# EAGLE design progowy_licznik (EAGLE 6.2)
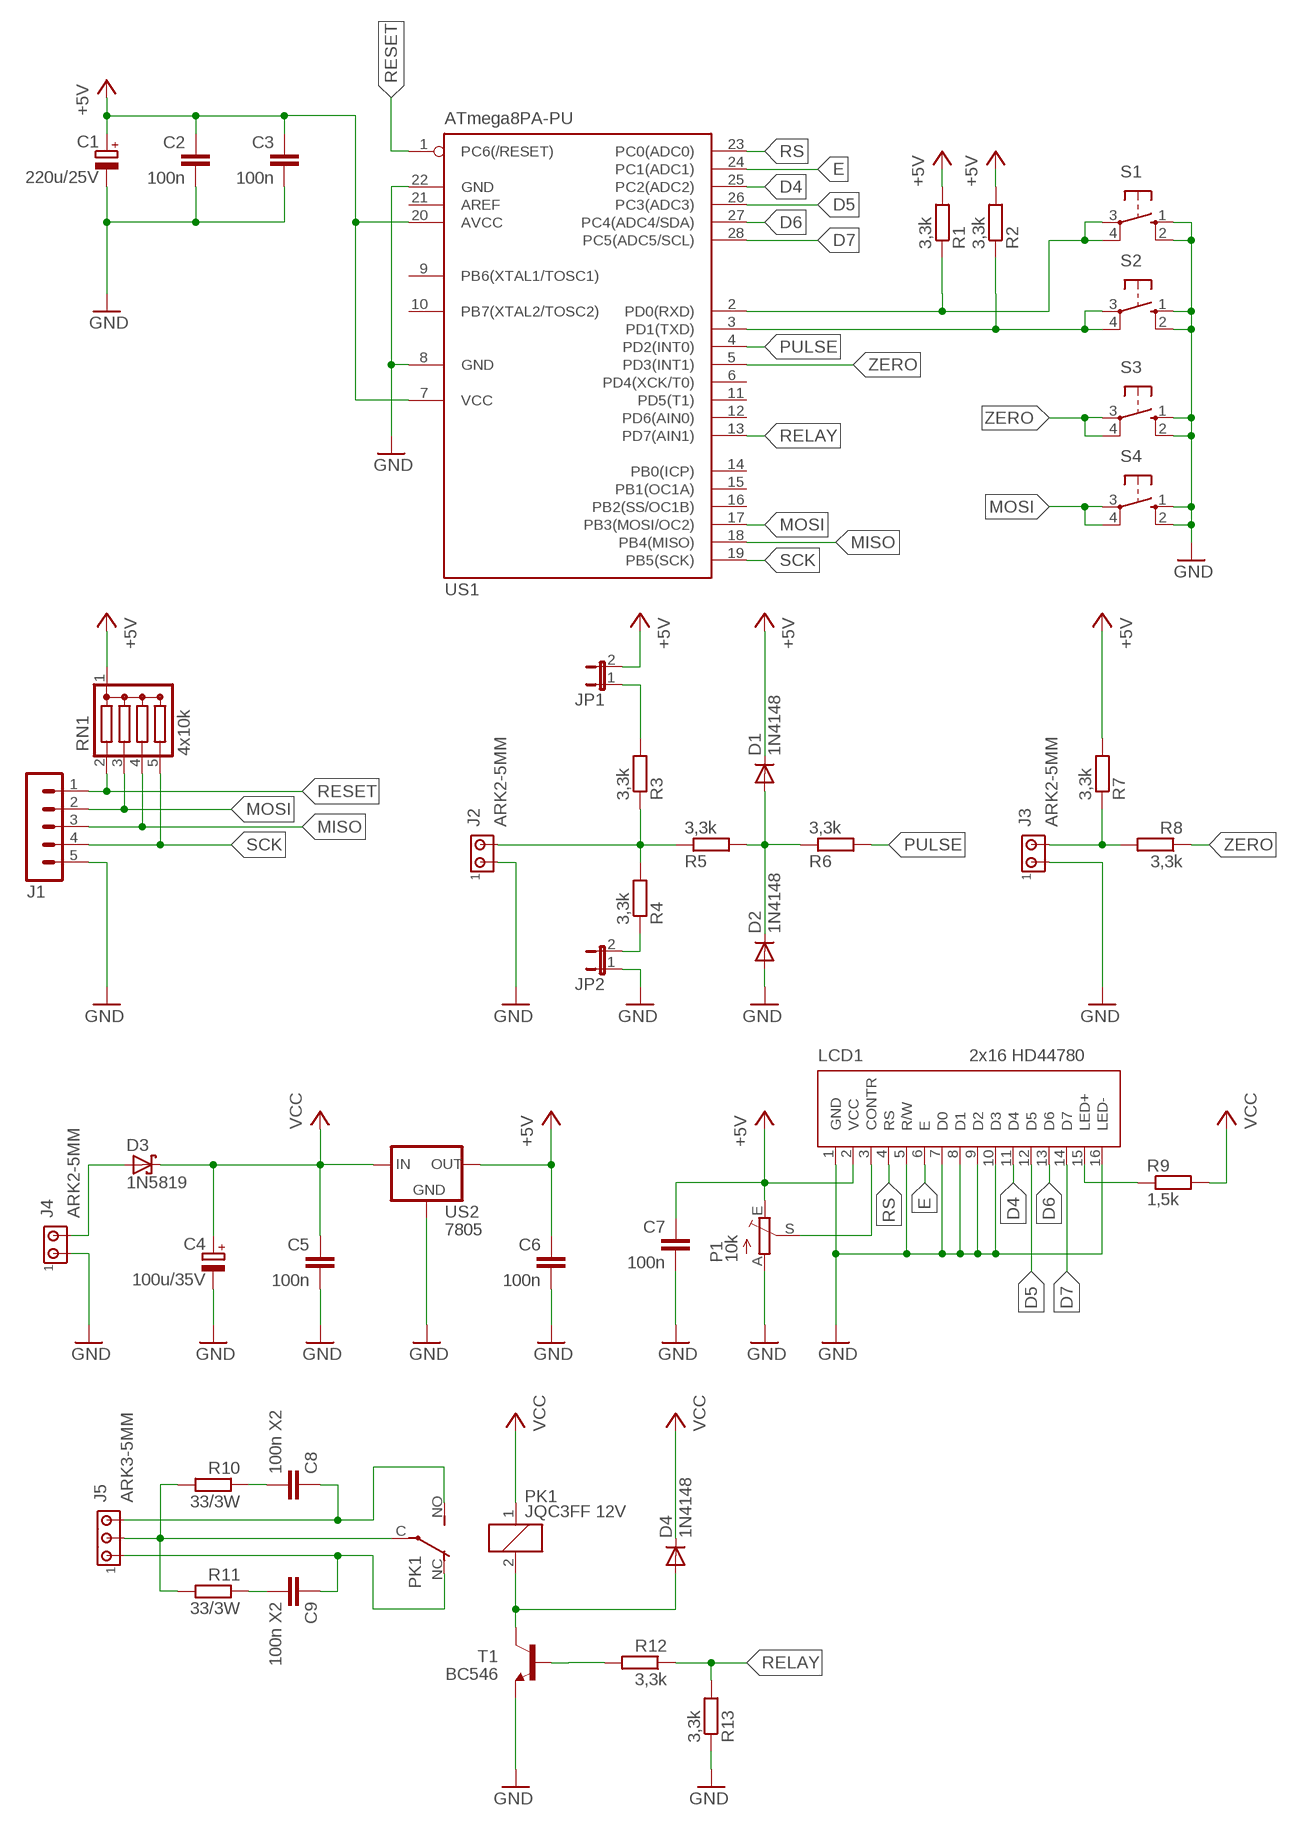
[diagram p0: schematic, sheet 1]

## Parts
C1  220u/25V  CPOL-EUE2.5-7  [E2,5-7]
C2  100n  C-EU050-025X075  [C050-025X075]
C3  100n  C-EU050-025X075  [C050-025X075]
C4  100u/35V  CPOL-EUE2.5-7  [E2,5-7]
C5  100n  C-EU050-025X075  [C050-025X075]
C6  100n  C-EU050-025X075  [C050-025X075]
C7  100n  C-EU050-025X075  [C050-025X075]
C8  100n X2  C-EU102_152-062X184  [C102_152-062X184]
C9  100n X2  C-EU102_152-062X184  [C102_152-062X184]
D1  1N4148  BAT81  [DO34-7]
D2  1N4148  BAT81  [DO34-7]
D3  1N5819  SCHOTTKY-DIODEF126Z12  [F126Z12]
D4  1N4148  BAT81  [DO34-7]
J1  MA05-1  [MA05-1]
J2  ARK2-5MM  [2PIN-5MM]
J3  ARK2-5MM  [2PIN-5MM]
J4  ARK2-5MM  [2PIN-5MM]
J5  ARK3-5MM  [3PIN-5MM]
JP1  JP1E  [JP1]
JP2  JP1E  [JP1]
LCD1  2x16 HD44780  LCD_2X16-NAD-ELEMENTAMI  [LCD_HD44780_2X16_NAD-ELEMENTAMI]
P1  10k  TRIM_EU-CA6V  [CA6V]
PK1  JQC3FF 12V  PK_POJED-JQC-3FG  [PK_POJED_JQC-3FG]
R1  3,3k  R-EU_0207/7  [0207/7]
R2  3,3k  R-EU_0207/7  [0207/7]
R3  3,3k  R-EU_0207/7  [0207/7]
R4  3,3k  R-EU_0207/7  [0207/7]
R5  3,3k  R-EU_0207/7  [0207/7]
R6  3,3k  R-EU_0207/7  [0207/7]
R7  3,3k  R-EU_0207/7  [0207/7]
R8  3,3k  R-EU_0207/7  [0207/7]
R9  1,5k  R-EU_0207/7  [0207/7]
R10  33/3W  R-EU_0617/17  [0617/17]
R11  33/3W  R-EU_0617/17  [0617/17]
R12  3,3k  R-EU_0207/7  [0207/7]
R13  3,3k  R-EU_0207/7  [0207/7]
RN1  4x10k  DRAB_REZ_1X4  [RN-5]
S1  10-XX  [B3F-10XX]
S2  10-XX  [B3F-10XX]
S3  10-XX  [B3F-10XX]
S4  10-XX  [B3F-10XX]
T1  BC546  BC546A  [TO92-EBC]
US1  ATmega8PA-PU  MEGA8-P  [DIL28-3]
US2  7805  78XXL  [78XXL]

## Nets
+5V: C1.+ C2.1 C3.1 C6.1 C7.1 D1.C JP1.2 LCD1.2(VCC) P1.E R1.2 R2.2 R7.2 RN1.1(C) US1.7(VCC) US1.20(AVCC) US2.OUT
D4: LCD1.11(D4) US1.25(PC2(ADC2))
D5: LCD1.12(D5) US1.26(PC3(ADC3))
D6: LCD1.13(D6) US1.27(PC4(ADC4/SDA))
D7: LCD1.14(D7) US1.28(PC5(ADC5/SCL))
E: LCD1.6(E) US1.24(PC1(ADC1))
GND: C1.- C2.2 C3.2 C4.- C5.2 C6.2 C7.2 D2.A J1.5 J2.P$1 J3.P$1 J4.P$1 JP2.1 LCD1.1(GND) LCD1.5(R/W) LCD1.7(D0) LCD1.8(D1) LCD1.9(D2) LCD1.10(D3) LCD1.16(LED-) P1.A R13.1 S1.1(S) S1.2(S1) S2.1(S) S2.2(S1) S3.1(S) S3.2(S1) S4.1(S) S4.2(S1) T1.E US1.8(GND) US1.22(GND) US2.GND
MISO: J1.3 RN1.4 US1.18(PB4(MISO))
MOSI: J1.2 RN1.3 S4.3(P) S4.4(P1) US1.17(PB3(MOSI/OC2))
N$1: LCD1.3(CONTR) P1.S
N$2: J5.P$2 PK1.C(COM) R10.2 R11.2
N$3: JP1.1 R3.2
N$4: JP2.2 R4.1
N$5: R1.1 S1.3(P) S1.4(P1) US1.2(PD0(RXD))
N$6: LCD1.15(LED+) R9.1
N$7: R12.2 T1.B
N$8: D3.A J4.P$2
N$9: D4.A PK1.2 T1.C
N$10: R2.1 S2.3(P) S2.4(P1) US1.3(PD1(TXD))
N$11: C8.1 J5.P$3 PK1.NO
N$12: C9.1 J5.P$1 PK1.NC
N$13: C8.2 R10.1
N$14: C9.2 R11.1
N$15: J3.P$2 R7.1 R8.2
N$20: J2.P$2 R3.1 R4.2 R5.1
N$21: D1.A D2.C R5.2 R6.1
PULSE: R6.2 US1.4(PD2(INT0))
RELAY: R12.1 R13.2 US1.13(PD7(AIN1))
RESET: J1.1 RN1.2 US1.1(PC6(/RESET))
RS: LCD1.4(RS) US1.23(PC0(ADC0))
SCK: J1.4 RN1.5 US1.19(PB5(SCK))
VCC: C4.+ C5.1 D3.C D4.C PK1.1 R9.2 US2.IN
ZERO: R8.1 S3.3(P) S3.4(P1) US1.5(PD3(INT1))
Unconnected: US1.6(PD4(XCK/T0)) US1.9(PB6(XTAL1/TOSC1)) US1.10(PB7(XTAL2/TOSC2)) US1.11(PD5(T1)) US1.12(PD6(AIN0)) US1.14(PB0(ICP)) US1.15(PB1(OC1A)) US1.16(PB2(SS/OC1B)) US1.21(AREF)

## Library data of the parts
C1 C4 = rcl:CPOL-EU: POLARIZED CAPACITOR, European symbol
C2 C3 C5-C9 = rcl:C-EU: CAPACITOR, European symbol
D1 D2 D4 = diode:BAT81: DIODE
D3 = diode:SCHOTTKY-DIODE: Schottky Diode
J1 = zlacza_futrzak:MA05-1: PIN HEADER; OC_FARNELL: unknown; OC_NEWARK: unknown
J2-J4 = zlacza_futrzak:ARK2: ARK 2
J5 = zlacza_futrzak:ARK3: ARK 3 Raster 5mm i 3,5mm
JP1 JP2 = jumper:JP1E: JUMPER
LCD1 = inne_futrzak:LCD_2X16
P1 = pot:TRIM_EU-: POTENTIOMETER
PK1 = inne_futrzak:PK_POJED
R1-R13 = rcl:R-EU_: RESISTOR, European symbol
RN1 = inne_futrzak:DRAB_REZ_1X4
S1-S4 = switch-omron:10-XX: OMRON SWITCH; MPN: B3F-1000; OC_FARNELL: 176432; OC_NEWARK: 36M3542
T1 = transistor-npn:BC546*: NPN Transistor
US1 = atmel:MEGA8-P: MICROCONTROLLER 8 Kbytes FLASH, 1 kbytes SRAM, 512 bytes EEPROM, USART, 4-channel 10 bit ADC, 2-channel 8 bit ADC Pin compatible with Atmega48, ATMega88, ATMega168 Source: avr.lbr; OC_FARNELL: unknown; OC_NEWARK: unknown
US2 = v-reg:78XXL: VOLTAGE REGULATOR

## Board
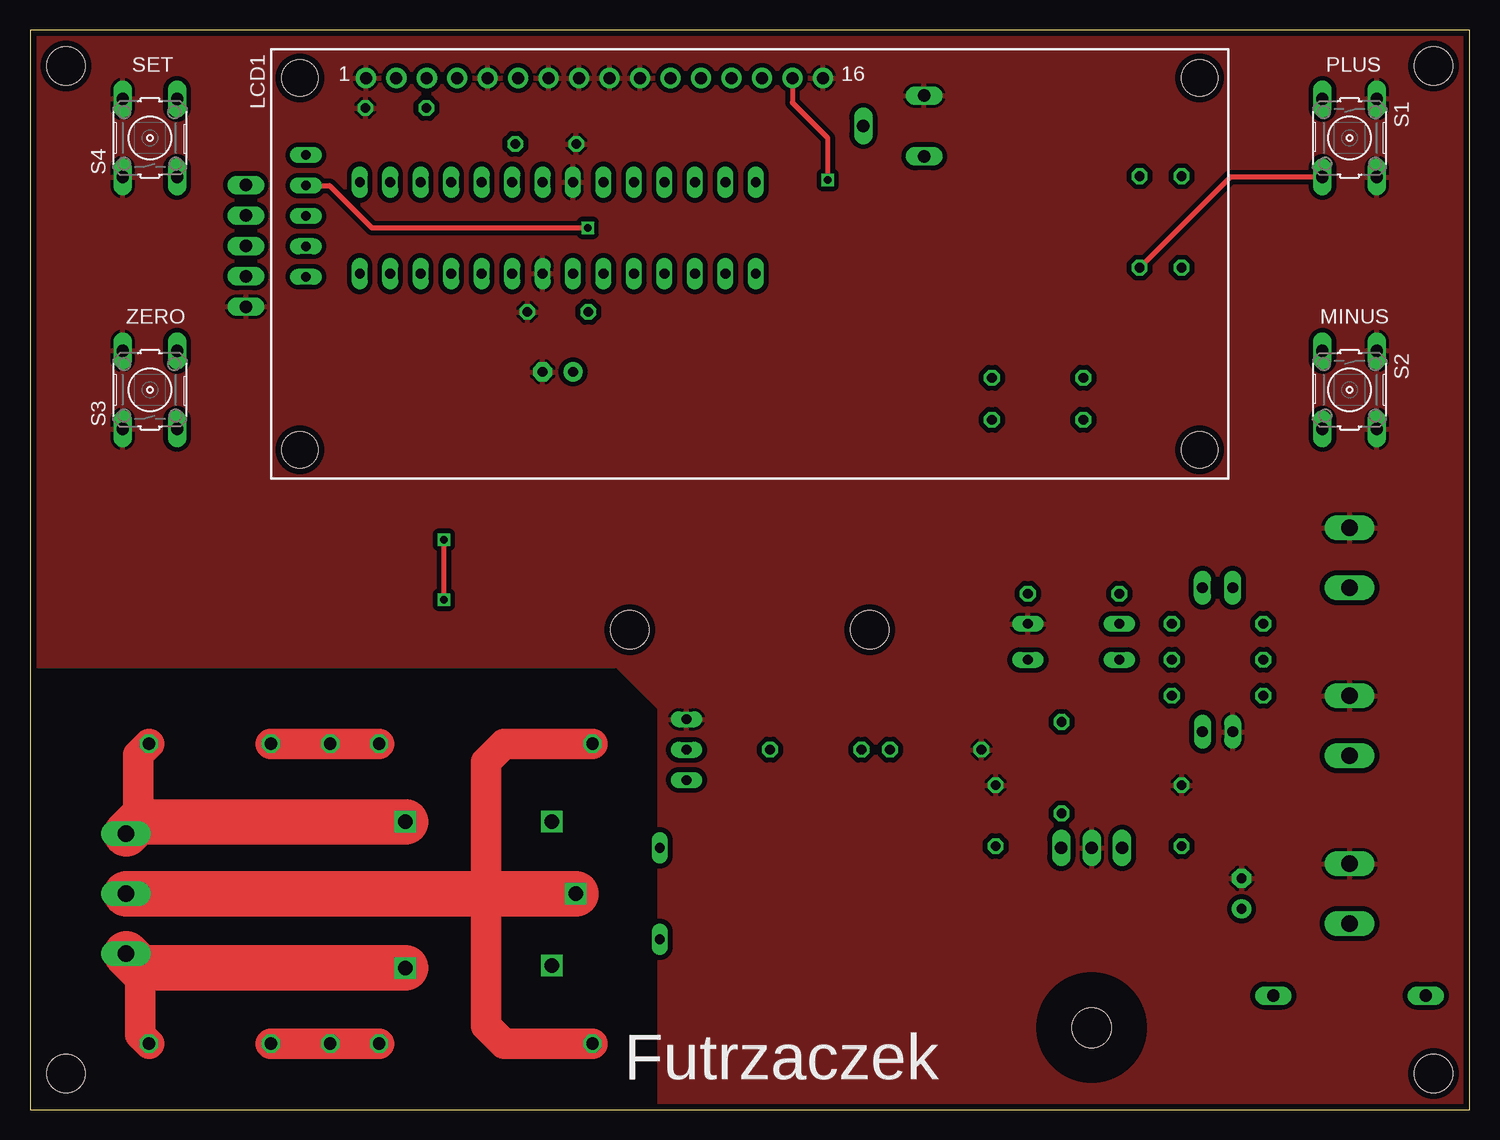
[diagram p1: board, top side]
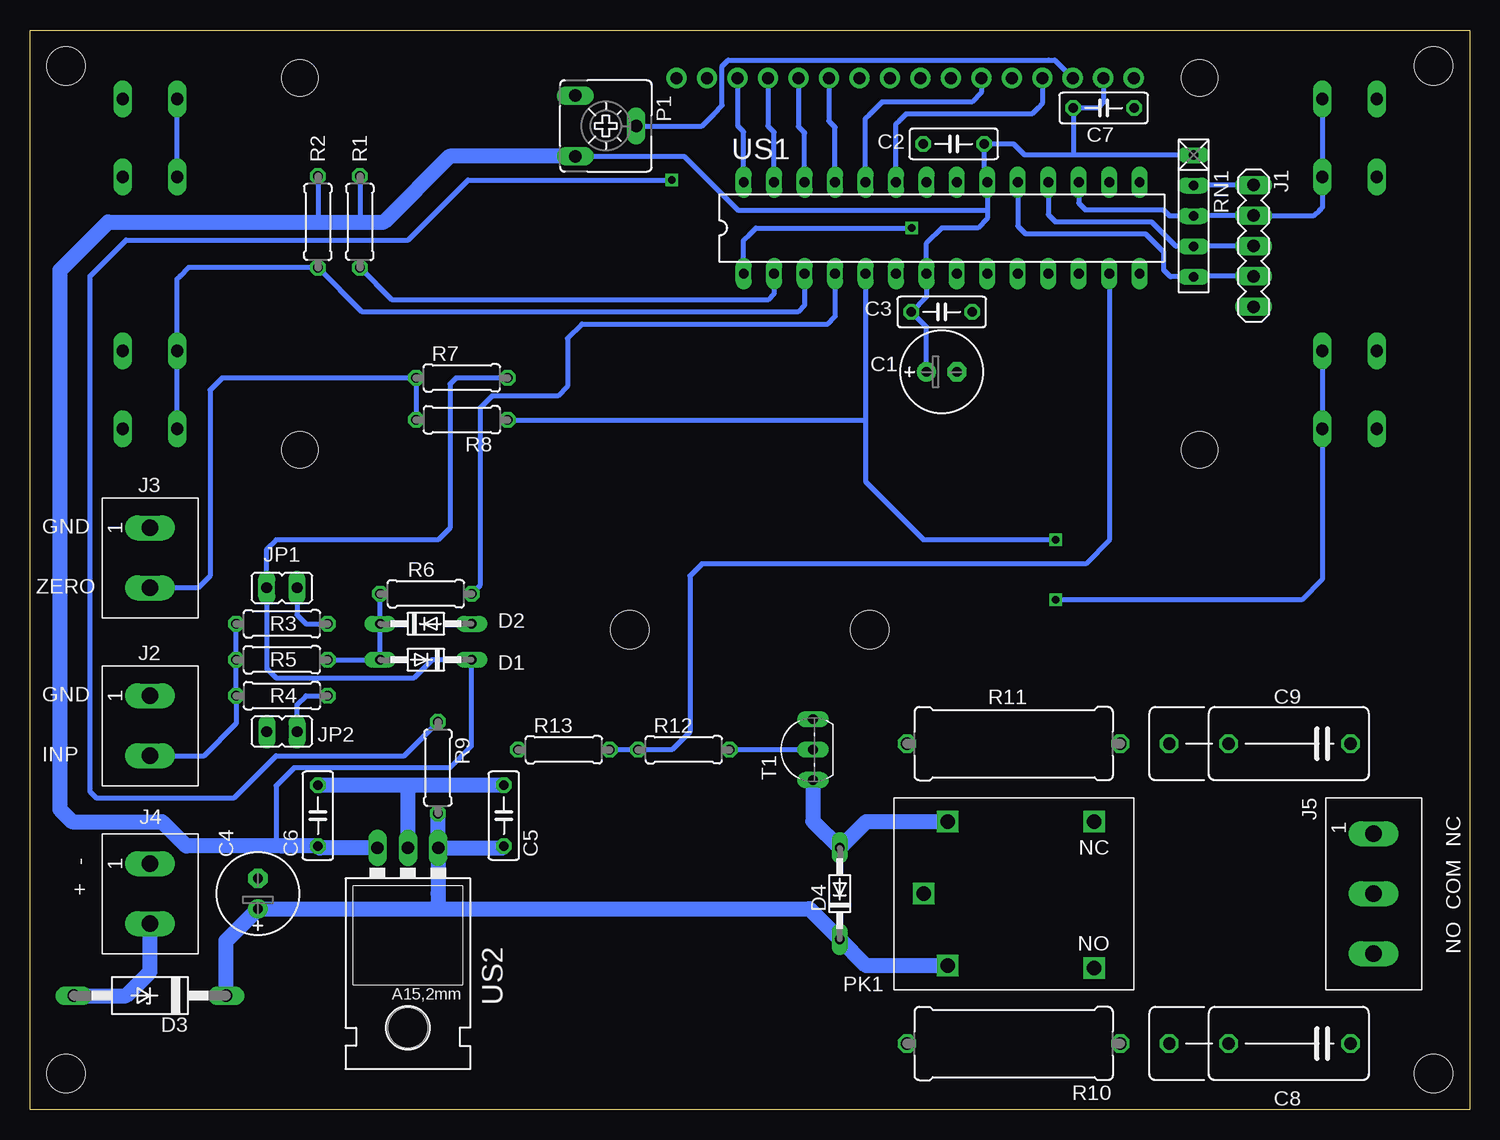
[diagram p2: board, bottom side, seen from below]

Size 120 x 90 mm. Coordinates in mm from the lower left corner, seen from the top.
Outline: 0,0 120,0 120,90 0,90 0,0
Copper layers (1*16): Top 0.035mm / dielectric 1.5mm / Bottom 0.035mm
Design rules: minimum track width 10mil, minimum drill 23mil, track to track 8mil, track to pad 8mil, pad to pad 8mil, via to via 8mil, smd to smd 8mil, copper to edge 20mil, drill to drill 8mil, minimum pad ring 10mil, minimum via ring 8mil, stop-mask expansion 4mil, vias tented up to drill 0mil, thermal gap 10mil
Holes 3.2 mm at 3,87 117,87 50,40 70,40 3,3 117,3

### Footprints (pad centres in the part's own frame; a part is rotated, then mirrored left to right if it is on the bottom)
E2,5-7 = drill 0.813 pad 1.6: + -1.27,0 | drill 0.813 pad 1.6 octagon: - 1.27,0
C050-025X075 = drill 0.813 octagon: 1 -2.54,0; 2 2.54,0
C102_152-062X184 = drill 1.016 octagon: 1 -5.08,0; 2 5.08,0; 3 10.033,0
DO34-7 = drill 0.813 long: A 3.81,0; C -3.81,0
F126Z12 = drill 1.016 long: A 6.35,0; C -6.35,0
MA05-1 = drill 1.016 long: 1 -5.08,0; 2 -2.54,0; 3 0,0; 4 2.54,0; 5 5.08,0
2PIN-5MM = drill 1.4 long: P$1 -2.5,0; P$2 2.5,0
3PIN-5MM = drill 1.4 long: P$1 -5,0; P$2 0,0; P$3 5,0
JP1 = drill 0.914 long: 1 0,-1.27; 2 0,1.27
LCD_HD44780_2X16_NAD-ELEMENTAMI = drill 1 pad 1.676: 1 -32,15.5; 2 -29.46,15.5; 3 -26.92,15.5; 4 -24.38,15.5; 5 -21.84,15.5; 6 -19.3,15.5; 7 -16.76,15.5; 8 -14.22,15.5; 9 -11.68,15.5; 10 -9.14,15.5; 11 -6.6,15.5; 12 -4.06,15.5; 13 -1.52,15.5; 14 1.02,15.5; 15 3.56,15.5; 16 6.1,15.5 | hole 3: -37.5,-15.5; 37.5,-15.5; -37.5,15.5; 37.5,15.5
CA6V = drill 1.016 long: A -2.54,-2.54; E 2.54,-2.54; S 0,2.54
PK_POJED_JQC-3FG = drill 1.2 square: 1 5.5,6; 2 5.5,-6; C 7.5,0; NC -6.7,-6; NO -6.7,6.2
0207/7 = drill 0.813 octagon: 1 -3.81,0; 2 3.81,0
0617/17 = drill 1.016 octagon: 1 -8.89,0; 2 8.89,0
RN-5 = drill 0.813 long: 1 -5.08,0; 2 -2.54,0; 3 0,0; 4 2.54,0; 5 5.08,0
B3F-10XX = drill 1.016 long: 1 -3.251,2.261; 2 3.251,2.261; 3 -3.251,-2.261; 4 3.251,-2.261
TO92-EBC = drill 0.813 long: B 0,-1.27; C -2.54,-1.27; E 2.54,-1.27
DIL28-3 = drill 0.813 long: 1 -16.51,-3.81; 2 -13.97,-3.81; 3 -11.43,-3.81; 4 -8.89,-3.81; 5 -6.35,-3.81; 6 -3.81,-3.81; 7 -1.27,-3.81; 8 1.27,-3.81; 9 3.81,-3.81; 10 6.35,-3.81; 11 8.89,-3.81; 12 11.43,-3.81; 13 13.97,-3.81; 14 16.51,-3.81; 15 16.51,3.81; 16 13.97,3.81; 17 11.43,3.81; 18 8.89,3.81; 19 6.35,3.81; 20 3.81,3.81; 21 1.27,3.81; 22 -1.27,3.81; 23 -3.81,3.81; 24 -6.35,3.81; 25 -8.89,3.81; 26 -11.43,3.81; 27 -13.97,3.81; 28 -16.51,3.81
78XXL = drill 1.016 long: GND 0,-3.81; IN -2.54,-3.81; OUT 2.54,-3.81 | hole 3.302: 0,11.176

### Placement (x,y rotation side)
C1  44,61.5 0 bottom
C2  43,80.5 180 bottom
C3  44,66.5 0 bottom
C4  101,18 90 bottom
C5  80.5,24.5 90 bottom
C6  96,24.5 90 bottom
C7  30.5,83.5 0 bottom
C8  15,5.5 180 bottom
C9  15,30.5 180 bottom
D1  87,37.5 180 bottom
D2  87,40.5 0 bottom
D3  110,9.5 180 bottom
D4  52.5,18 90 bottom
J1  18,72 270 bottom
J2  110,32 270 bottom
J3  110,46 270 bottom
J4  110,18 270 bottom
J5  8,18 270 bottom
JP1  99,43.5 90 bottom
JP2  99,31.5 270 bottom
LCD1  60,70.5 0 top
P1  72,82 270 bottom
PK1  38,18 180 bottom
R1  92.5,74 90 bottom
R2  96,74 90 bottom
R3  99,40.5 0 bottom
R4  99,34.5 180 bottom
R5  99,37.5 0 bottom
R6  87,43 0 bottom
R7  84,61 0 bottom
R8  84,57.5 180 bottom
R9  86,28.5 270 bottom
R10  38,5.5 180 bottom
R11  38,30.5 180 bottom
R12  65.5,30 0 bottom
R13  75.5,30 0 bottom
RN1  23,74.5 270 bottom
S1  110,81 270 top
S2  110,60 270 top
S3  10,60 90 top
S4  10,81 90 top
T1  56,30 90 bottom
US1  44,73.5 0 bottom
US2  88.5,18 180 bottom

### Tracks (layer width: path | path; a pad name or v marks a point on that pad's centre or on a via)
+5V
  Bottom 0.406: 40.19,75 US1.20 40.46,77.58 C2.1 38,80.5 37.08,79.58 33,79.58 | 40.19,75 40.19,74.31 41,73.5 44,73.5 45.27,72.23 US1.7 45.27,67.77 C3.1 45.27,65.23 C1.+ | RN1.1 33,79.58 | 33,79.58 33.04,79.62 C7.1 31,83.5 30.54,83.96 LCD1.2 | 40.19,75 61,75 65.46,79.46 P1.E | 99,21.96 99.5,22.46 99.5,27 98,28.5 85,28.5 83.19,30.31 D1.C 86.5,37.5 88,36 99.5,36 100.27,36.77 JP1.2 100.27,46.73 99.5,47.5 86,47.5 85,48.5 85,60.5 84.5,61 R7.2 | R1.2 92.5,74 | R2.2 96,74
  Bottom 1.27: US2.OUT 95.85,21.81 C6.1 99,21.96 106.96,21.96 109,24 116.5,24 117.5,25 117.5,70 113.5,74 96,74 92.5,74 90.5,74 85.04,79.46 P1.E
D4
  Bottom 0.406: US1.25 52.89,81.89 53,82 53.4,82.4 LCD1.11
D5
  Bottom 0.406: US1.26 55.43,81.43 55.94,81.94 LCD1.12
D6
  Bottom 0.406: US1.27 57.97,81.47 58.48,81.98 LCD1.13
D7
  Bottom 0.406: US1.28 60.51,81.51 61,82 61.02,82.02 LCD1.14
E
  Bottom 0.406: LCD1.6 40.7,84.8 41.5,84 49,84 50,83 50.35,82.65 US1.24
GND
  Bottom 1.27: C5.2 88.5,27.04 | 88.5,27.04 C6.2 | US2.GND 88.5,27.04
  pour Top (isolate 0.406): 0,90 120,90 120,0 52.5,0 52.5,17 52.5,33.5 49,37 0,37
MISO
  Bottom 0.406: J1.3 22.96,72 RN1.4 24.46,71.96 26.5,74 34.5,74 35.11,74.61 US1.18
MOSI
  Bottom 0.406: US1.17 32.57,75.57 32,75 25.5,75 25,74.5 RN1.3 22.96,74.54 J1.2 12.96,74.54 12.5,75 12.26,75.24 S4.3 S4.4
N$1
  Bottom 0.406: P1.S 64,82 63,83 62.3,83.7 62.3,87 61.8,87.5 35.08,87.5 34.58,87.5 LCD1.3
N$2
  Top 2.54: R11.2 39.5,30.5 38,29 38,18 | R10.2 39.5,5.5 38,7 38,17.5 37.5,18
  Top 3.81: PK1.C 38,18 37.5,18 J5.P$2
N$3
  Bottom 0.406: JP1.1 97.73,41.23 97,40.5 R3.2
N$4
  Bottom 0.406: JP2.2 97.73,33.77 97,34.5 R4.1
N$5
  Top 0.406: S1.4 100.06,77.75 R1.1
  Bottom 0.406: S1.4 S1.3 | US1.2 57.97,68.03 58.5,67.5 89.81,67.5 R1.1
N$6  (via drill 0.6)
  Top 0.406: v66.5,77.5 66.5,81 63.56,83.94 LCD1.15
  Bottom 0.406: v66.5,77.5 83.5,77.5 88.5,72.5 112,72.5 115,69.5 115,26.5 114.5,26 103,26 99.5,29.5 88.81,29.5 R9.1
N$7
  Bottom 0.406: T1.B R12.2
N$8
  Bottom 1.27: D3.A 112,9.5 110,11.5 J4.P$2
N$9
  Bottom 1.27: PK1.2 50.31,24 D4.A 54.73,24.04 T1.C
N$10
  Bottom 0.406: S2.4 S2.3 107.74,69.26 107.5,69.5 106.81,70.19 R2.1 92.31,66.5 56,66.5 55.43,67.07 US1.3
N$11
  Top 2.54: 9.2,11.8 9.2,6.22 C8.1
  Top 3.81: PK1.NO 9.2,11.8 J5.P$3
N$12
  Top 2.54: 9,24 9,29.58 C9.1
  Top 3.81: PK1.NC 9,24 J5.P$1
N$13
  Top 2.54: C8.2 R10.1
N$14
  Top 2.54: C9.2 R11.1
N$15
  Bottom 0.406: J3.P$2 106,43.5 105,44.5 105,60 104,61 R7.1 R8.2
N$20
  Bottom 0.406: J2.P$2 105.5,29.5 102.81,32.19 R4.2 R5.1 R3.1
N$21
  Bottom 0.406: R5.2 D1.A D2.C R6.1
PULSE
  Bottom 0.406: US1.4 52.89,66.11 53.5,65.5 74,65.5 75.19,64.31 75.19,60.31 76,59.5 81.5,59.5 82.5,58.5 82.5,43.69 R6.2
RELAY
  Bottom 0.406: R13.2 R12.1 66.5,30 65,31.5 65,44.5 64,45.5 32,45.5 30.03,47.47 US1.13
RESET  (via drill 0.6)
  Top 0.406: v46.5,73.5 28.5,73.5 26,76 24.96,77.04 RN1.2
  Bottom 0.406: J1.1 22.96,77.08 RN1.2 | US1.1 60.51,72.49 60,73 59.5,73.5 v46.5,73.5
RS
  Bottom 0.406: LCD1.4 35.62,83.88 36,83.5 36.5,83 47,83 47.5,82.5 47.81,82.19 US1.23
SCK
  Bottom 0.406: J1.4 22.96,69.46 RN1.5 23.92,69.42 24.92,69.42 25.5,70 25.5,71.5 26.5,72.5 27,73 37,73 37.5,73.5 37.65,73.65 US1.19
VCC
  Bottom 1.27: D3.C 103.65,14.08 C4.+ 86,16.73 | US2.IN 85.96,18.04 86,18 86,16.73 | US2.IN 80.65,21.81 C5.1 | US2.IN 85.96,24.65 R9.2 | 86,16.73 55.04,16.73 D4.C 50.31,12 PK1.1
ZERO  (via drill 0.6)
  Top 0.406: v34.5,42.5 v34.5,47.5
  Bottom 0.406: R8.1 50.35,57.5 | US1.5 50.35,57.5 | 50.35,57.5 50.35,52.35 45.5,47.5 v34.5,47.5 | v34.5,42.5 14,42.5 12.26,44.24 S3.3 S3.4

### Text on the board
tPlace: SET | PLUS | ZERO | MINUS | Futrzaczek
bPlace: GND | ZERO | GND | INP | NO COM NC | + -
